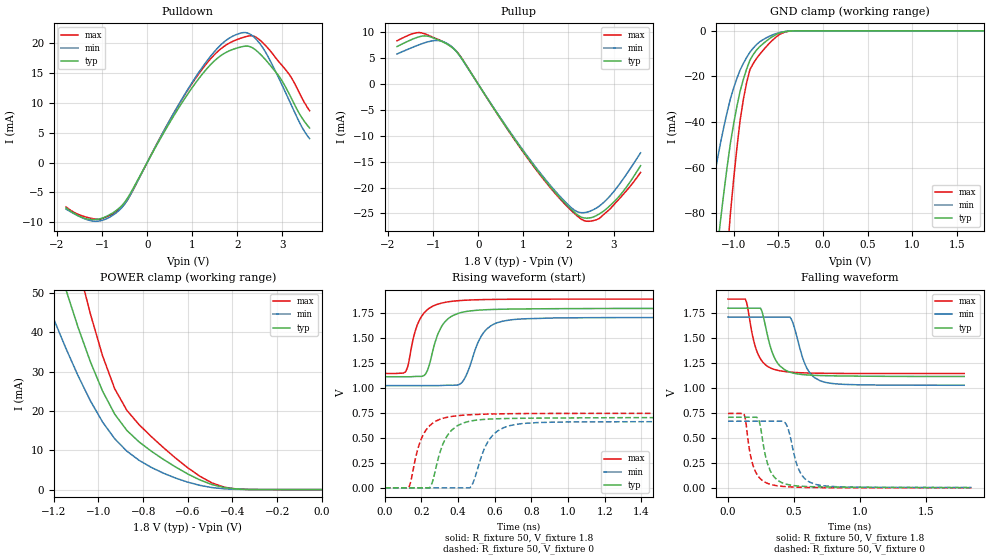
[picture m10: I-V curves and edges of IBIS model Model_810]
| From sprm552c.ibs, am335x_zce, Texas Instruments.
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| Model based on original model for BCSHTLTCSCDDVPBFZ_SSDHV
|   Sub model SR00_5MA_PADN_5PER_1P8
[model]   Model_810
|[Description]  [1.8V-3-STATE-NOTERM-SR00:5MA, IND, 5%]
|   Fastest slew rate (SR[1:0] = "00"), 1.60 * RExt = 0.625 * Iout
|   (I[2:0] = "000"), 5mA nominal with Rext = 50R,ODT off (ODT[1:0]
|   = "00") CMOS mode,Industrial temperature range (-40C to 125C,
|   25C nominal),5% power supply tolerance
|[Input Load]   NOTERM
|[Output Drive] SR00:5MA
|Voltage   1.8V
|Mode   3-STATE
Model_type   3-state
Polarity   Non-Inverting
Enable   Active-Low
Cref =  15pF
Rref =  100.0000M
Vref =  0V
Vmeas =  0.9
C_comp   1.851324p   1.667199p   1.973575p
[Temperature Range]   25   125   -40
[Voltage Range]   1.8   1.71   1.89
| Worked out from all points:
|   slope of the pulldown table from 0 to 0.27 V, typ, clamps not added: 72.9 ohm
|   slope of the pullup table from 0 to 0.27 V, typ, clamps not added: 73.8 ohm
|   GND clamp passes 1 mA (typ) near -0.49 V on its own axis
|   POWER clamp passes 1 mA (typ) near -0.47 V on its own axis
|   rising waveform, R_fixture 50, V_fixture 1.8: 20-80 % time 81.3ps typ, 93.5ps min, 75.4ps max; typ from 1.11 V to 1.8 V
|   rising waveform, R_fixture 50, V_fixture 0: 20-80 % time 86.1ps typ, 94.1ps min, 81ps max; typ from 0 V to 0.703 V
|   falling waveform, R_fixture 50, V_fixture 1.8: 20-80 % time 97.3ps typ, 104ps min, 87.7ps max; typ from 1.8 V to 1.11 V
|   falling waveform, R_fixture 50, V_fixture 0: 20-80 % time 80.1ps typ, 87.9ps min, 72.1ps max; typ from 0.707 V to 0.003 V
[POWER_clamp]
-1.8V     194.9mA    137mA      262.9mA
-1.236V   68.49mA    48.49mA    92.7mA
-1.145V   50.76mA    35.84mA    69.67mA
-1.127V   47.56mA    33.52mA    65.35mA
-1.055V   35.4mA     24.68mA    48.7mA
-981.8mV  25.06mA    17.19mA    34.02mA
-927.3mV  19.17mA    12.92mA    25.62mA
-872.7mV  15.03mA    9.76mA     20.13mA
-818.2mV  12.12mA    7.445mA    16.51mA
-654.5mV  5.738mA    2.929mA    8.007mA
-436.4mV  508.2uA    199.4uA    613uA
0V        2.273nA    16.6nA     10.58nA
[Pulldown]
-1.8V     -7.609mA   -7.815mA   -7.446mA
-1.145V   -9.551mA   -9.863mA   -9.487mA
-600mV    -7.505mA   -7.866mA   -7.717mA
-381.8mV  -5.292mA   -5.559mA   -5.572mA
490.9mV   6.589mA    6.96mA     6.97mA
1.091V    13.54mA    14.52mA    14.32mA
1.636V    17.95mA    19.77mA    19.1mA
2.073V    19.37mA    21.71mA    20.85mA
2.291V    19.41mA    21.49mA    21.27mA
2.564V    17.74mA    19.25mA    20.08mA
3.164V    11.28mA    10.17mA    14.61mA
3.6V      5.787mA    4.008mA    8.697mA
[Pullup]
-1.8V     7.273mA    5.836mA    8.384mA
-1.2V     9.332mA    7.957mA    9.779mA
-872.7mV  8.52mA     8.421mA    8.6mA
-600mV    7.23mA     7.34mA     7.272mA
-381.8mV  5.181mA    5.112mA    5.231mA
1.2V      -15.41mA   -15.19mA   -15.57mA
1.8V      -21.85mA   -21.57mA   -22.06mA
2.182V    -25.16mA   -24.61mA   -25.39mA
2.4V      -25.92mA   -24.79mA   -26.51mA
2.673V    -25.16mA   -23.66mA   -26.04mA
3.164V    -21.3mA    -18.96mA   -21.84mA
3.6V      -15.77mA   -13.28mA   -17.07mA
[GND_clamp]
-1.8V     -346.1mA   -209.3mA   -568.3mA
-1.327V   -149.7mA   -89.03mA   -250.9mA
-1.291V   -135.6mA   -80.47mA   -227.5mA
-1.145V   -82.35mA   -48.67mA   -137.7mA
-1.073V   -59.44mA   -35.55mA   -97.96mA
-1.036V   -49.1mA    -29.72mA   -79.9mA
-927.3mV  -26.31mA   -17.11mA   -38.99mA
-854.5mV  -16.67mA   -11.64mA   -22.56mA
-818.2mV  -12.86mA   -9.351mA   -16.98mA
-672.7mV  -5.705mA   -3.913mA   -8.623mA
-381.8mV  -120.4uA   -129uA     -167.2uA
1.8V      2.273nA    51.44nA    6.654nA
[Ramp]
dV/dt_f 0.41859457/98.760477p 0.41916117/0.10503421n 0.45116787/87.772717p
dV/dt_r 0.42891327/87.257311p 0.40631124/94.62713p  0.45121837/80.91337p
R_load = 50
[Rising Waveform]
R_fixture = 50
V_fixture = 1.8
V_fixture_min = 1.71
V_fixture_max = 1.89
0s        1.113V     1.024V     1.146V
114.7ps   1.113V     1.024V     1.168V
169.3ps   1.116V     1.024V     1.59V
216ps     1.128V     1.024V     1.755V
283.9ps   1.513V     1.024V     1.836V
314ps     1.629V     1.026V     1.852V
421.4ps   1.758V     1.056V     1.877V
527.3ps   1.781V     1.524V     1.885V
645.9ps   1.789V     1.67V      1.888V
1.787ns   1.797V     1.705V     1.89V
[Rising Waveform]
R_fixture = 50
V_fixture = 0
V_fixture_min = 0
V_fixture_max = 0
0s        0V         0V         0V
128.7ps   0V         0V         0V
187.2ps   0V         0V         432.2mV
244.4ps   0V         0V         621.6mV
302ps     362.2mV    0V         687.3mV
336.5ps   510.3mV    0V         705.5mV
464.1ps   667.9mV    0V         732mV
569.4ps   688.7mV    482.1mV    739.2mV
686.1ps   695.2mV    624.9mV    742.8mV
1.842ns   703.1mV    662.9mV    746.1mV
[Falling Waveform]
R_fixture = 50
V_fixture = 1.8
V_fixture_min = 1.71
V_fixture_max = 1.89
0s        1.799V     1.71V      1.89V
130.5ps   1.799V     1.71V      1.89V
145ps     1.799V     1.71V      1.83V
198.4ps   1.799V     1.71V      1.451V
245.7ps   1.799V     1.71V      1.291V
349.1ps   1.309V     1.71V      1.186V
468.9ps   1.158V     1.71V      1.159V
594.1ps   1.131V     1.205V     1.15V
701.4ps   1.124V     1.07V      1.147V
1.787ns   1.115V     1.027V     1.145V
[Falling Waveform]
R_fixture = 50
V_fixture = 0
V_fixture_min = 0
V_fixture_max = 0
0s        706.9mV    667.2mV    745.1mV
121.4ps   706.9mV    667.2mV    736.5mV
177ps     706.9mV    667.2mV    283.8mV
231.1ps   684mV      667.2mV    111.8mV
284.4ps   313.3mV    667.2mV    53.75mV
321.4ps   166.6mV    667.2mV    34.93mV
439.5ps   37.35mV    637.9mV    11.94mV
531.2ps   18.35mV    196mV      6.355mV
647.1ps   11.15mV    40.9mV     3.207mV
1.842ns   2.681mV    4.291mV    0V
